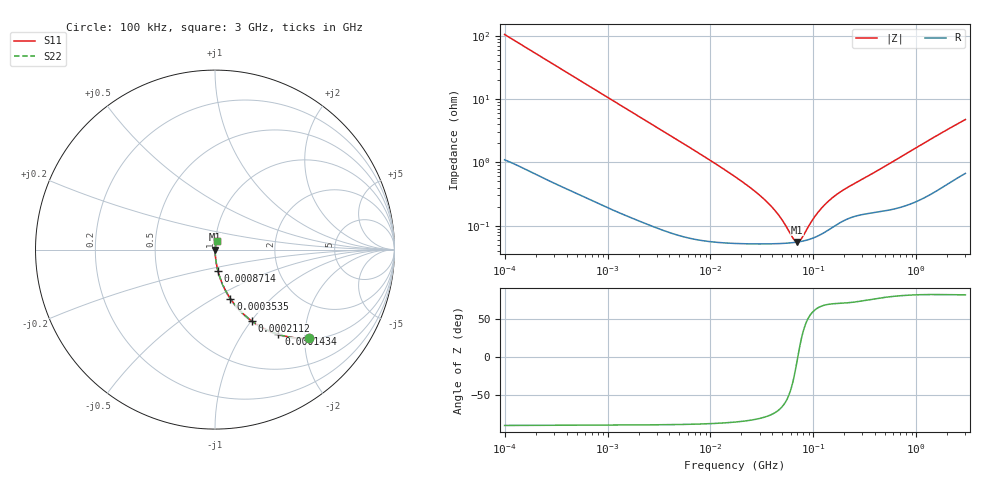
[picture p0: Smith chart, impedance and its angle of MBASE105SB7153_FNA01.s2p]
! MBASE105SB7153_FNA01  S-PARAMETER MODEL  ( Standard Model )
! Model Generated by TAIYO YUDEN Corporation (http://www.ty-top.com)
! Version 1.0
! TAIYO YUDEN Control No. 220601
! Copyright(c) 2017 TAIYO YUDEN CO.,LTD. All Rights Reserved.
! Product Description (link to TY-COMPAS)
! https://ds.yuden.co.jp/TYCOMPAS/or/detail?pn=MBASE105SB7153KFNA01&u=M
! Products Name : Multilayer Ceramic Capacitors
! Characteristics :
!  Capacitance : 0.015 [uF] , Rated Voltage : 16 [V] , TCC : X7R
!  Case Size : 1.0 x 0.5 / 0.039 x 0.02 [mm/inch] , Thickness : 0.5 / 0.02 [mm/inch]
!  (Conditions: Temperature = 25 [degC] , DC Bias Voltage = 0 [V])
! External Node Assignments :
!  1  o---| |---o  2
! GND o---------o GND
! Frequency Range : 100kHz  -  3GHz  [ 401 STEP ]
# MHZ S RI R 50
! Freq[MHz].  S11 Real  S11 Imag  S21 Real  S21 Imag  S12 Real  S12 Imag  S22 Real  S22 Imag
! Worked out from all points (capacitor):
!   401 points, 100 kHz to 3 GHz, reference 50 ohm
!   read as one part in series: C = 15.1 nF near 105.3 kHz
!   lowest |Z| = 55.2 mohm at 69.66 MHz (marker M1)
!   series resonance near 70.5 MHz, so ESL is about 340 pH
!   S11 on the Smith chart (normalised r, x): 100 kHz: 1.02, -2.11; 143.4 kHz: 1.02, -1.47; 211.2 kHz: 1.01, -1.00; 353.5 kHz: 1.01, -0.60; 871.4 kHz: 1.00, -0.25; 3 GHz: 1.01, +0.09
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0.1  0.5256 -0.4941  0.4744 0.4941  0.4744 0.4941  0.5256 -0.4941
0.14345  0.3532 -0.4722  0.6468 0.4722  0.6468 0.4722  0.3532 -0.4722
0.21115  0.204 -0.3968  0.796 0.3968  0.796 0.3968  0.204 -0.3968
0.353547  0.0862 -0.2737  0.9138 0.2737  0.9138 0.2737  0.0862 -0.2737
0.562235  0.0375 -0.1822  0.9625 0.1822  0.9625 0.1822  0.0375 -0.1822
0.871356  0.0169 -0.1207  0.9831 0.1207  0.9831 0.1207  0.0169 -0.1207
1.576268  0.00603 -0.0679  0.994 0.0679  0.994 0.0679  0.00603 -0.0679
3.161081  0.00206 -0.0342  0.9979 0.0342  0.9979 0.0342  0.00206 -0.0342
17.7727  0.000556 -0.00576  0.9994 0.00576  0.9994 0.00576  0.000556 -0.00576
27.54426  0.000526 -0.00337  0.9995 0.00337  0.9995 0.00337  0.000526 -0.00337
38.50681  0.00052 -0.002  0.9995 0.002  0.9995 0.002  0.00052 -0.002
48.55934  0.000524 -0.00119  0.9995 0.00119  0.9995 0.00119  0.000524 -0.00119
64.47533  0.000541 -0.00028  0.9995 0.00028  0.9995 0.00028  0.000541 -0.00028
69.65816  0.00055 -3.73e-05  0.9994 3.73e-05  0.9994 3.73e-05  0.00055 -3.73e-05
73.34282  0.000558 0.000125  0.9994 -0.000125  0.9994 -0.000125  0.000558 0.000125
77.22239  0.000566 0.000287  0.9994 -0.000287  0.9994 -0.000287  0.000566 0.000287
97.38194  0.00063 0.00103  0.9994 -0.00103  0.9994 -0.00103  0.00063 0.00103
126.0104  0.000772 0.00191  0.9992 -0.00191  0.9992 -0.00191  0.000772 0.00191
167.3121  0.00104 0.00291  0.999 -0.00291  0.999 -0.00291  0.00104 0.00291
547.5153  0.00185 0.00936  0.9981 -0.00936  0.9981 -0.00936  0.00185 0.00936
1658.39  0.00446 0.0273  0.9955 -0.0273  0.9955 -0.0273  0.00446 0.0273
3000  0.00884 0.0465  0.9912 -0.0465  0.9912 -0.0465  0.00884 0.0465
